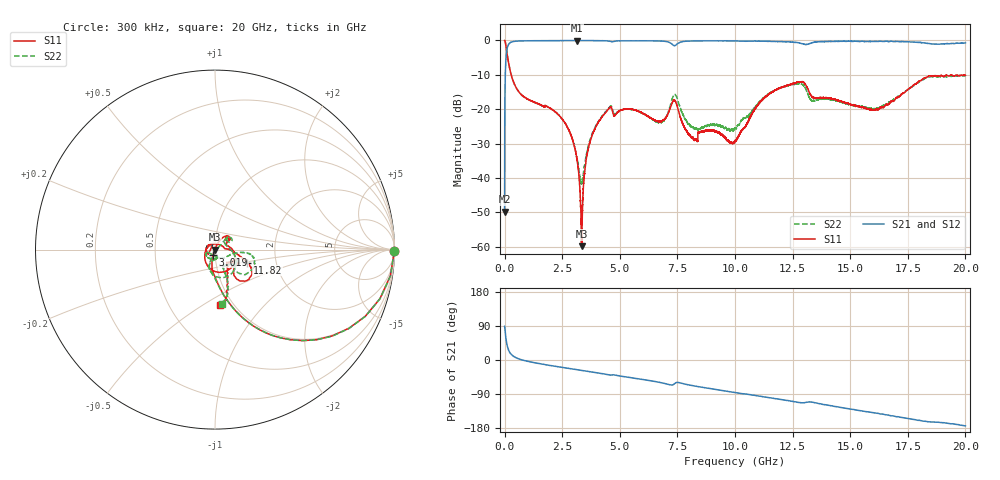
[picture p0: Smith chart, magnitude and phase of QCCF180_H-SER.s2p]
!{QCCF180}
!Johanson Technology Inc.
!www.johansontechnology.com
!Test Board Conditions:
!Substrate Type  RO4350B
!Substrate Thickness  10 mil
!Substrate Dk  3.66
!TL Type: GCPW
!TL Trace Width  21 mil
!TL Gap  20 mil
!Electrode orientation  Horizontal
!DUT TOPOLOGY	SERIES
!Mounting Pad LxW  16x21 mil
! Created Sat Jan  9 18:21:12 2021
# hz S ma R 50
! 2 Port Network Data from SP1.SP block
! freq  magS11  angS11  magS21  angS21  magS12  angS12  magS22  angS22
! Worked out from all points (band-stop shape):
!   20001 points, 300 kHz to 20 GHz, reference 50 ohm
!   highest |S21| = -0.03 dB at 3.156 GHz (marker M1); lowest = -49.8 dB at 300 kHz (marker M2)
!   |S21| within 3 dB of the highest: 91.47 MHz to end of sweep
!   lowest |S11| = -59.8 dB at 3.341 GHz (marker M3), VSWR 1.00, Z = 49.9 + j0.00157 ohm
!   |S11| at or under -10 dB: 285.3 MHz to end of sweep
!   |S22| runs from -41.8 to 0.0 dB; largest |S21 - S12| = 0.012
!   S11 on the Smith chart (normalised r, x): 300 kHz: open; 3.019 GHz: 0.98, -0.05; 11.82 GHz: 1.42, -0.21; 20 GHz: 0.87, -0.59
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300000  0.9992 -0.5  0.00325 89.2  0.003355 89.6  0.9989 -0.5
1.043e8  0.6565 -49.9  0.7503 39.9  0.7513 39.8  0.6574 -49.9
2.083e8  0.4078 -68.1  0.9104 21.4  0.9093 21.5  0.407 -68.2
6.493e8  0.1737 -87.0  0.983 2.3  0.9825 2.3  0.1731 -88.1
2.3103e9  0.08463 -101.7  0.993 -17.7  0.9942 -17.7  0.08418 -111.1
3.0193e9  0.02959 -110.0  0.9952 -24.4  0.9962 -24.4  0.03008 -106.1
3.1563e9  0.01714 -113.7  0.997 -25.7  0.9959 -25.8  0.01815 -95.9
3.3343e9  0.001431 -157.7  0.996 -27.3  0.9961 -27.4  0.008327 -34.1
3.3413e9  0.001022 179.1  0.9961 -27.4  0.9966 -27.5  0.008267 -31.1
3.5333e9  0.01791 70.0  0.9948 -29.3  0.9961 -29.3  0.02044 29.8
3.7123e9  0.03391 67.3  0.9948 -31.0  0.9953 -30.9  0.03593 38.8
4.5013e9  0.1006 50.1  0.9833 -38.8  0.9836 -38.8  0.1019 41.8
6.6673e9  0.06634 25.0  0.9833 -58.3  0.9833 -58.4  0.06426 33.5
7.3903e9  0.1338 -66.9  0.8398 -61.8  0.8412 -61.9  0.1652 -67.0
8.1713e9  0.03918 137.9  0.9818 -67.8  0.9835 -67.8  0.05484 -85.9
1.00003e10  0.03458 61.9  0.9851 -85.9  0.9827 -86.0  0.05327 -65.6
1.18163e10  0.1942 -21.8  0.9657 -102.5  0.9663 -102.6  0.1933 -7.3
1.28453e10  0.249 -37.5  0.9089 -112.7  0.9101 -112.7  0.2351 -28.6
1.33343e10  0.1533 -47.4  0.9216 -111.1  0.9229 -111.2  0.1326 -35.5
1.66673e10  0.1179 -54.6  0.9632 -145.5  0.9666 -145.9  0.1257 -66.6
1.83983e10  0.3025 -80.5  0.9039 -163.0  0.9062 -162.9  0.2939 -80.6
2e10  0.3104 -84.8  0.9216 -174.0  0.9181 -173.9  0.3075 -83.4
